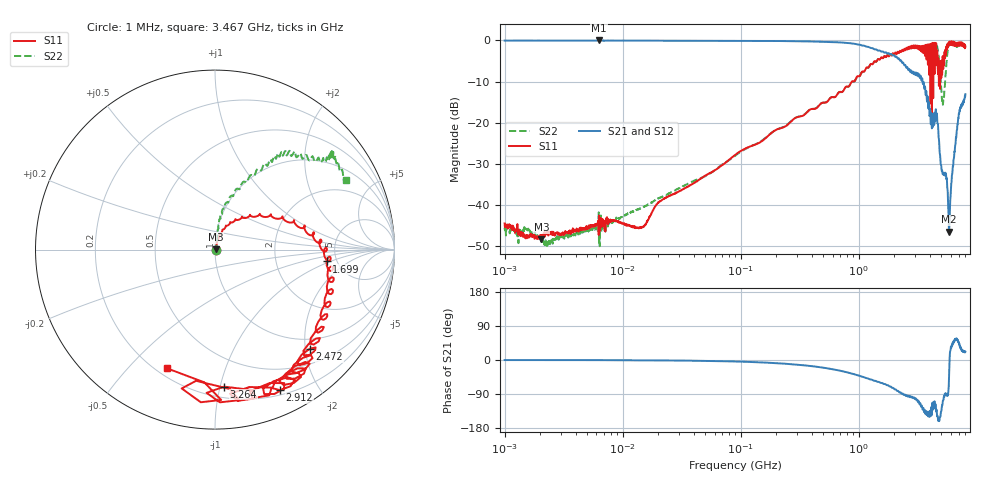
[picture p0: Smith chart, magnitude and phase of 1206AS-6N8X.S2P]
!s-Parameter Generated by FASTRON Sdn. Bhd.
!FASTRON P/N : 1206AS-6N8X
!Keysight Technologies: E5071C_MY46733604_B.14.02
!Date: Wed Nov 15 09:31:49 2023
!Version  :Rev00  Wed Nov 15 09:31:49 2023
!Data & Calibration Information:
!Freq  S11:SOLT2(ON)  S21:SOLT2(ON)  S12:SOLT2(ON)  S22:SOLT2(ON)
!PortZ  Port1:50+j0  Port2:50+j0
!When reading reference impedance value at option line is always used.
! Remarks : This data is being provided solely for informational purposes.
# Hz S dB R 50
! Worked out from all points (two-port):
!   1601 points, 1 MHz to 8 GHz, reference 50 ohm
!   highest |S21| = -0.01 dB at 6.301 MHz (marker M1); lowest = -46.5 dB at 5.808 GHz (marker M2)
!   |S21| within 3 dB of the highest: start of sweep to 1.716 GHz
!   lowest |S11| = -48.4 dB at 2.048 MHz (marker M3), VSWR 1.01, Z = 50.4 + j0.0763 ohm
!   |S11| at or under -10 dB: start of sweep to 873.3 MHz; 4.043 GHz to 4.067 GHz (23.5 MHz wide, 0.579 % of centre); 4.143 GHz to 4.181 GHz (38.58 MHz wide, 0.927 % of centre)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
!   |S22| runs from -50.1 to -0.5 dB; largest |S21 - S12| = 0.0069
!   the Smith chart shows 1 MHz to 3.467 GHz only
!   S11 on the Smith chart (normalised r, x): 1 MHz: 1.01, -0.00; 1.699 GHz: 4.13, -0.90; 2.472 GHz: 0.79, -2.09; 2.912 GHz: 0.25, -1.53; 3.264 GHz: 0.28, -1.03; 3.467 GHz: 0.24, -0.65
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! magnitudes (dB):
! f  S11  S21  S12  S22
! 1 MHz  -44.5  0.0  0.0  -45.6
! 2.048 MHz  -48.4  0.0  0.0  -48.1
! 4.479 MHz  -45.7  0.0  0.0  -47.0
! 6.301 MHz  -42.6  0.0  -0.1  -49.3
! 14.49 MHz  -45.5  0.0  -0.1  -40.7
! 20.07 MHz  -39.4  -0.1  -0.1  -38.5
! 89.95 MHz  -27.8  -0.1  -0.1  -28.0
! 400.7 MHz  -16.7  -0.3  -0.3  -16.7
! 1.699 GHz  -4.1  -2.9  -2.9  -4.0
! 1.795 GHz  -3.9  -3.1  -3.1  -3.8
! 2.472 GHz  -2.3  -6.0  -6.0  -2.4
! 2.912 GHz  -1.3  -8.2  -8.2  -1.4
! 3.264 GHz  -2.3  -8.3  -8.3  -1.6
! 3.467 GHz  -2.9  -9.8  -9.8  -1.7
! 4.095 GHz  -2.3  -19.4  -19.4  -1.3
! 4.521 GHz  -0.6  -18.6  -18.6  -0.9
! 4.884 GHz  -11.8  -27.9  -27.9  -8.0
! 5.164 GHz  -5.6  -32.4  -32.4  -15.7
! 5.808 GHz  -0.4  -46.5  -46.6  -0.9
! 6.034 GHz  -0.6  -36.2  -36.2  -0.6
! 7.036 GHz  -1.3  -17.8  -17.8  -1.3
! 8 GHz  -1.5  -13.1  -13.1  -1.1
